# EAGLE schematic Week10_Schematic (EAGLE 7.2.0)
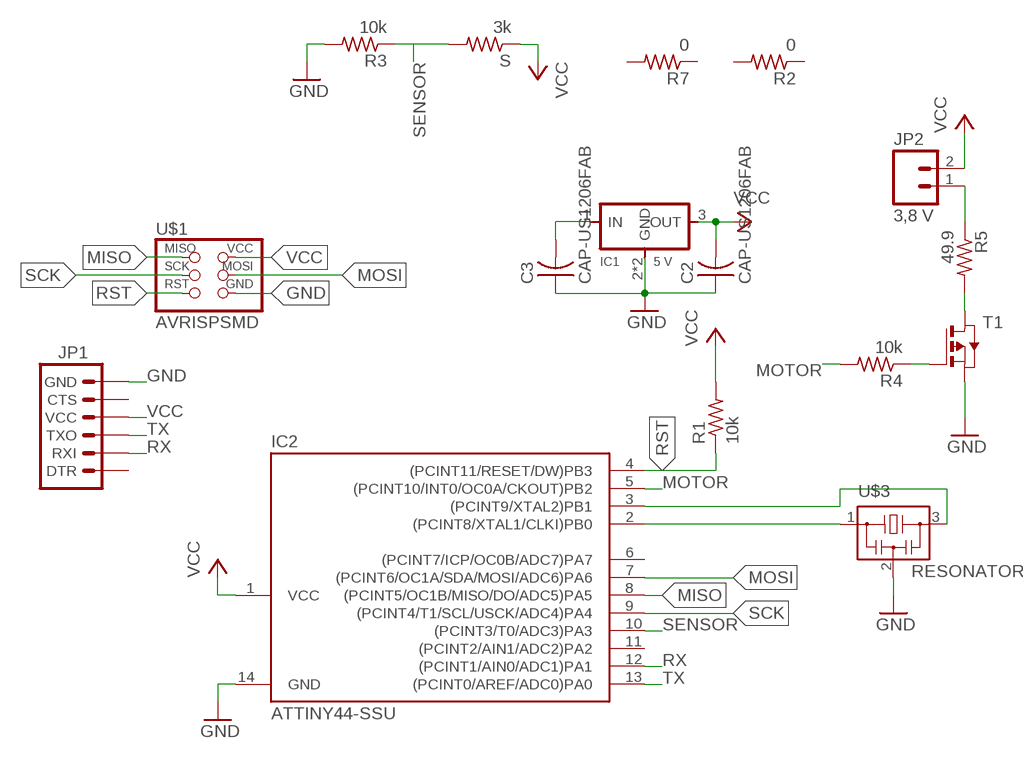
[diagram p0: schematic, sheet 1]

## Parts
C2  CAP-US1206FAB  [C1206FAB]
C3  CAP-US1206FAB  [C1206FAB]
IC1  5 V  REGULATORSOT223  [SOT223]
IC2  ATTINY44-SSU  [SOIC14]
JP1  ARDUINO_SERIAL_PROGRAMSMD  [1X06-SMD]
JP2  3,8 V  M023.5MM_LOCK  [SCREWTERMINAL-3.5MM-2_LOCK]
R1  10k  RES-US1206FAB  [R1206FAB]
R2  0  RES-US1206FAB  [R1206FAB]
R3  10k  RES-US1206FAB  [R1206FAB]
R4  10k  RES-US1206FAB  [R1206FAB]
R5  49.9  RES-US1206FAB  [R1206FAB]
R7  0  RES-US1206FAB  [R1206FAB]
S  3k  RES-US1206FAB  [R1206FAB]
T1  PMOSFETSOT23  [SOT-23]
U$1  AVRISPSMD  [2X03SMD]
U$3  RESONATOR  [EFOBM]

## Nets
GND: C2.1 C3.1 IC1.2(GND) IC1.4(GND) IC2.14(GND) JP1.6(GND) R3.2 T1.2(S) U$1.6(GND) U$3.2
MISO: IC2.8((PCINT5/OC1B/MISO/DO/ADC5)PA5) U$1.1(MISO)
MOSI: IC2.7((PCINT6/OC1A/SDA/MOSI/ADC6)PA6) U$1.4(MOSI)
MOTOR: IC2.5((PCINT10/INT0/OC0A/CKOUT)PB2) R4.2
N$1: JP2.1 R5.1
N$2: R5.2 T1.1(D)
N$3: IC2.2((PCINT8/XTAL1/CLKI)PB0) U$3.1
N$4: IC2.3((PCINT9/XTAL2)PB1) U$3.3
N$7: C3.2 IC1.1(IN)
N$8: R4.1 T1.3(G)
RST: IC2.4((PCINT11/RESET/DW)PB3) R1.1 U$1.5(RST)
RX: IC2.12((PCINT1/AIN0/ADC1)PA1) JP1.2(RXI)
SCK: IC2.9((PCINT4/T1/SCL/USCK/ADC4)PA4) U$1.3(SCK)
SENSOR: IC2.10((PCINT3/T0/ADC3)PA3) R3.1 S.2
TX: IC2.13((PCINT0/AREF/ADC0)PA0) JP1.3(TXO)
VCC: C2.2 IC1.3(OUT) IC2.1(VCC) JP1.4(VCC) JP2.2 R1.2 S.1 U$1.2(VCC)
Unconnected: IC2.6((PCINT7/ICP/OC0B/ADC7)PA7) IC2.11((PCINT2/AIN1/ADC2)PA2) JP1.1(DTR) JP1.5(CTS) R2.1 R2.2 R7.1 R7.2

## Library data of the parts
C2 C3 = 01_fab:CAP-US
IC1 = 01_fab:REGULATOR
IC2 = 01_fab:ATTINY44
JP1 = SparkFun-Connectors:ARDUINO_SERIAL_PROGRAM: FTDI connector footprints
JP2 = SparkFun-Connectors:M02: Standard 2-pin 0.1" header. Use with; PROD_ID: CONN-08399
R1-R5 R7 S = 01_fab:RES-US: Resistor (US Symbol)
T1 = 01_fab:PMOSFET: MOS FET
U$1 = fab:AVRISP
U$3 = 01_fab:RESONATOR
